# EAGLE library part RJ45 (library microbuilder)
RJ45 (Ethernet) Connectors J0026D21BNL - RJ45 Connector with internal transformer and 2 LEDs (Yellow/Green). LEDs have max foreward-voltage of 2.5V. LEDs require an external resistor. Digikey: 553-1349-ND J00-0065NL - RJ45 Connector with internal transformer and 2 LEDs (Yellow/Green). LEDs have max foreward-voltage of 2.5V. LEDs require an external resistor. Digikey: 553-1345-ND
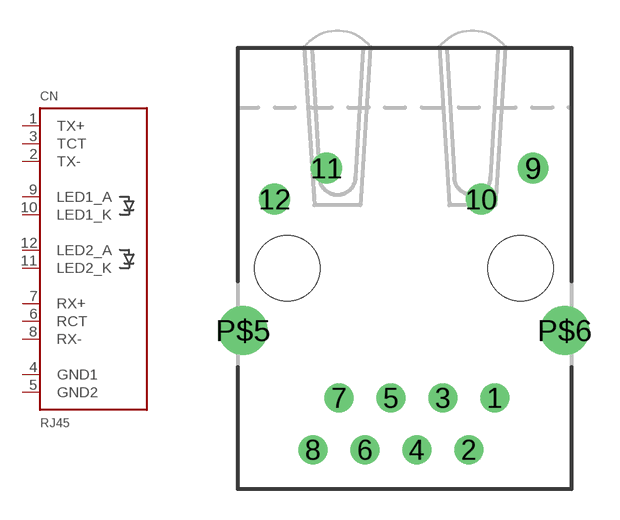
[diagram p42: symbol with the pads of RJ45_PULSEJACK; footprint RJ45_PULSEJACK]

Designator prefix CN

## RJ45J0026D21BNL  [RJ45_PULSEJACK]
1  TX+
2  TX-
3  TCT
4  GND1
5  GND2
6  RCT
7  RX+
8  RX-
9  LED1_A
10  LED1_K
11  LED2_K
12  LED2_A

## RJ45J000065NL  [RJ45_PULSEJACK]
1  TX+
2  TX-
3  RX+
4  TCT
5  RCT
6  RX-
7  GND2
8  GND1
9  LED1_A
10  LED1_K
11  LED2_K
12  LED2_A

## Footprint RJ45_PULSEJACK (pad centres in mm)
RJ45 (Ethernet) Connector with LEDs and Built-In Transformer Model: J0026D21BNL Digikey: 553-1349-ND
drill 0.9: 1 4.445,-6.35; 2 3.175,-8.89; 3 1.905,-6.35; 4 0.635,-8.89; 5 -0.635,-6.35; 6 -1.905,-8.89; 7 -3.175,-6.35; 8 -4.445,-8.89
drill 1: 9 6.325,4.9; 10 3.785,3.38; 11 -3.785,4.9; 12 -6.325,3.38
drill 1.6: P$5 -7.875,-3.05; P$6 7.875,-3.05
hole 3.2 at -5.715,0
hole 3.2 at 5.715,0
